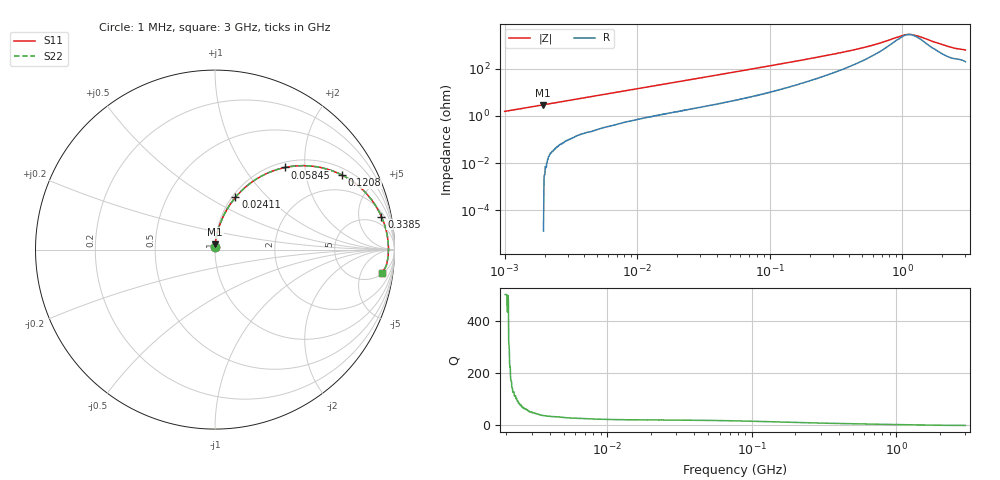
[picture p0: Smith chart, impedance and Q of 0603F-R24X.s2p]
!s-Parameter Generated by FASTRON Sdn. Bhd.
!FASTRON P/N : 0603F-R24X
!Keysight Technologies: E4991B_MY54100416_A.01.15
!Date: Thu Jun 20 13:16:32 2024
!Version  :Rev00  Thu Jun 20 13:16:32 2024
!Data & Calibration Information:
!Freq  S11  S21  S12  S22
!PortZ  Port1:50+j0  Port2:50+j0
!When reading reference impedance value at option line is always used.
! Remarks : This data is being provided solely for informational purposes.
# Hz S dB R 50
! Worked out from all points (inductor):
!   1601 points, 1 MHz to 3 GHz, reference 50 ohm
!   read as one part in series: L = 245 nH near 1.041 MHz
!   highest Q = 229 at 1.946 MHz (marker M1), where L = 241 nH
!   self-resonance near 1.13 GHz
!   S11 on the Smith chart (normalised r, x): 1 MHz: 1.00, +0.03; 24.11 MHz: 1.04, +0.67; 58.45 MHz: 1.10, +1.58; 120.8 MHz: 1.27, +3.23; 338.5 MHz: 2.72, +9.42; 3 GHz: 5, -12
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1000000  -36.10 93.2  0.01 -0.9  0.01 -0.9  -36.10 93.2
1945520  -30.60 88.3  -0.00 -1.7  -0.00 -1.7  -30.60 88.3
3804036  -25.00 85.0  -0.03 -3.2  -0.03 -3.2  -25.00 85.0
7741750  -19.10 81.0  -0.10 -6.3  -0.10 -6.3  -19.10 81.0
1.447069e7  -14.10 75.6  -0.27 -11.4  -0.27 -11.4  -14.10 75.6
2.41077e7  -10.10 68.7  -0.60 -18.1  -0.60 -18.1  -10.10 68.7
3.652005e7  -7.19 60.8  -1.16 -25.9  -1.16 -25.9  -7.19 60.8
5.504702e7  -4.72 51.0  -2.17 -35.4  -2.17 -35.4  -4.72 51.0
5.845373e7  -4.41 49.5  -2.37 -36.9  -2.37 -36.9  -4.41 49.5
8.422788e7  -2.80 39.7  -3.88 -46.3  -3.88 -46.3  -2.80 39.7
1.207609e8  -1.71 30.3  -5.90 -54.9  -5.90 -54.9  -1.71 30.3
2.083556e8  -0.82 18.7  -9.84 -64.6  -9.84 -64.6  -0.82 18.7
3.385367e8  -0.49 11.2  -14.10 -68.5  -14.10 -68.5  -0.49 11.2
5.445776e8  -0.35 6.0  -19.20 -65.8  -19.20 -65.8  -0.35 6.0
7.925923e8  -0.31 2.7  -24.70 -52.2  -24.70 -52.2  -0.31 2.7
1.02815e9  -0.29 0.7  -29.00 -20.4  -29.00 -20.4  -0.29 0.7
1.10276e9  -0.29 0.2  -29.50 -5.6  -29.50 -5.6  -0.29 0.2
1.171007e9  -0.30 -0.3  -29.40 8.0  -29.40 8.0  -0.30 -0.3
1.347129e9  -0.30 -1.3  -27.80 32.7  -27.80 32.7  -0.30 -1.3
1.738771e9  -0.33 -3.4  -23.20 56.1  -23.20 56.1  -0.33 -3.4
2.289646e9  -0.40 -6.0  -19.10 63.1  -19.10 63.1  -0.40 -6.0
3e9  -0.52 -8.1  -16.50 63.2  -16.50 63.2  -0.52 -8.1
